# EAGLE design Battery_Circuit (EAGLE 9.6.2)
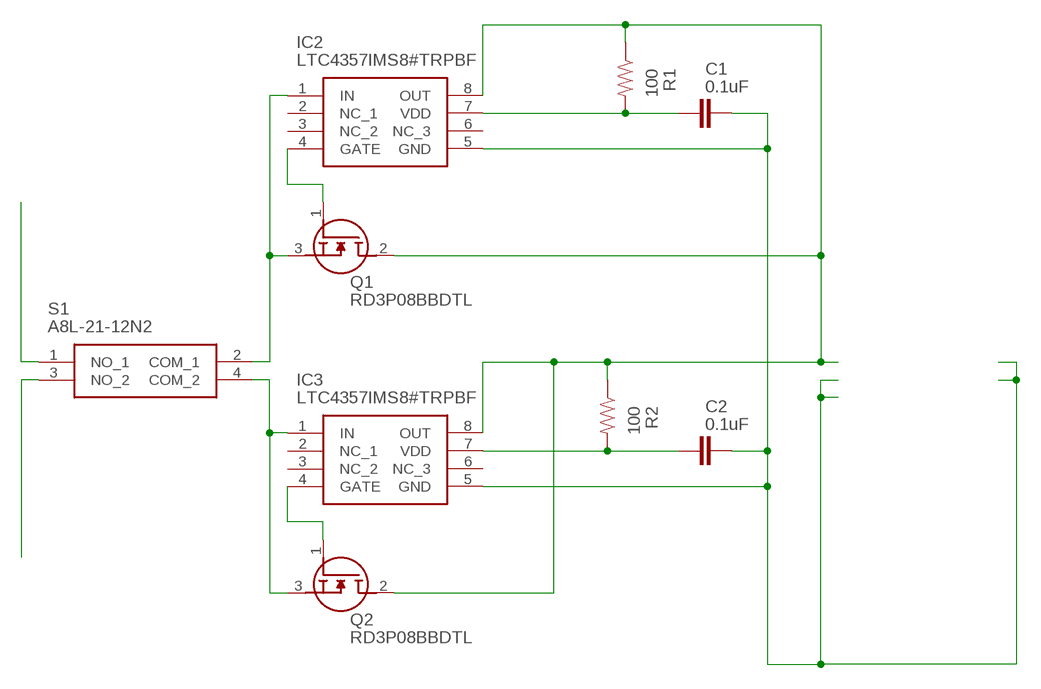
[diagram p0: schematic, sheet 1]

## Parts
C1  0.1uF  0.1UF-KIT-EZ-50V-20%  [CAP-PTH-SMALL-KIT]
C2  0.1uF  0.1UF-KIT-EZ-50V-20%  [CAP-PTH-SMALL-KIT]
IC2  LTC4357IMS8#TRPBF  [SOP65P490X110-8N]
IC3  LTC4357IMS8#TRPBF  [SOP65P490X110-8N]
Q1  RD3P08BBDTL  [RD3P175SNFRATL]
Q2  RD3P08BBDTL  [RD3P175SNFRATL]
R1  100  100OHM-HORIZ-1/4W-1%  [AXIAL-0.3]
R2  100  100OHM-HORIZ-1/4W-1%  [AXIAL-0.3]
S1  A8L-21-12N2  [A8L2112N2]

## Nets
N$1: IC2.1(IN) Q1.3(S) S1.2(COM_1)
N$2: IC2.4(GATE) Q1.1(G)
N$3: IC3.4(GATE) Q2.1(G)
N$4: S1.3(NO_2)
N$5: IC3.1(IN) Q2.3(S) S1.4(COM_2)
N$6: S1.1(NO_1)
N$7: C1.2 C2.2 IC2.5(GND) IC3.5(GND)
N$9: C1.1 IC2.7(VDD) R1.P$2
N$10: C2.1 IC3.7(VDD) R2.P$2
N$11: IC2.8(OUT) IC3.8(OUT) Q1.2(D) Q2.2(D) R1.P$1 R2.P$1
Unconnected: IC2.2(NC_1) IC2.3(NC_2) IC2.6(NC_3) IC3.2(NC_1) IC3.3(NC_2) IC3.6(NC_3)

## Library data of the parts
C1 C2 = SparkFun-Capacitors:0.1UF: 0.1µF ceramic capacitors; PROD_ID: CAP-08370
IC2 IC3 = SamacSys_Parts:LTC4357IMS8#TRPBF: Hot Swap Controller 1-CH 80V N-Channel Positive High Voltage Automotive 8-Pin MSOP T/R Source: Datasheet; ARROW_PART_NUMBER: LTC4357IMS8#TRPBF; ARROW_PRICE-STOCK: https://www.arrow.com/en/products/ltc4357ims8trpbf/analog-devices?region=nac; DESCRIPTION: Hot Swap Controller 1-CH 80V N-Channel Positive High Voltage Automotive 8-Pin MSOP T/R; HEIGHT: 1.1mm; MANUFACTURER_NAME: Analog Devices; MANUFACTURER_PART_NUMBER: LTC4357IMS8#TRPBF; MOUSER_PART_NUMBER: 584-LTC4357IMS8TRPBF; MOUSER_PRICE-STOCK: https://www.mouser.co.uk/ProductDetail/Analog-Devices/LTC4357IMS8TRPBF?qs=hVkxg5c3xu9xOCu4lpdF5Q%3D%3D
Q1 Q2 = SamacSys_Parts:RD3P08BBDTL: RD3P08BBDTL N-Channel MOSFET, 80 A, 100 V RD3P08BBD, 3-Pin DPAK ROHM Source: Datasheet; DESCRIPTION: RD3P08BBDTL N-Channel MOSFET, 80 A, 100 V RD3P08BBD, 3-Pin DPAK ROHM; HEIGHT: mm; MANUFACTURER_NAME: ROHM Semiconductor; MANUFACTURER_PART_NUMBER: RD3P08BBDTL; MOUSER_PART_NUMBER: 755-RD3P08BBDTL; MOUSER_PRICE-STOCK: https://www.mouser.co.uk/ProductDetail/ROHM-Semiconductor/RD3P08BBDTL?qs=qSfuJ%252Bfl%2Fd6NkJEicmek1A%3D%3D
R1 R2 = SparkFun-Resistors:100OHM: 100Ω resistor; PROD_ID: RES-12181
S1 = SamacSys_Parts:A8L-21-12N2: Rocker Switches ROCKER SWITCH Source: Datasheet; DESCRIPTION: Rocker Switches ROCKER SWITCH; HEIGHT: 22.1mm; MANUFACTURER_NAME: Omron Electronics; MANUFACTURER_PART_NUMBER: A8L-21-12N2; MOUSER_PART_NUMBER: 653-A8L-21-12N2; MOUSER_PRICE-STOCK: https://www.mouser.co.uk/ProductDetail/Omron-Electronics/A8L-21-12N2?qs=wE98CiVmOw76dmZWfHCJ3A%3D%3D

## Module DEWALT12V
Ports: 

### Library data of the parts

## Module 12V-5V_CONVERTER
Ports: IN-(in) IN+(in) OUT-(out) OUT+(out)

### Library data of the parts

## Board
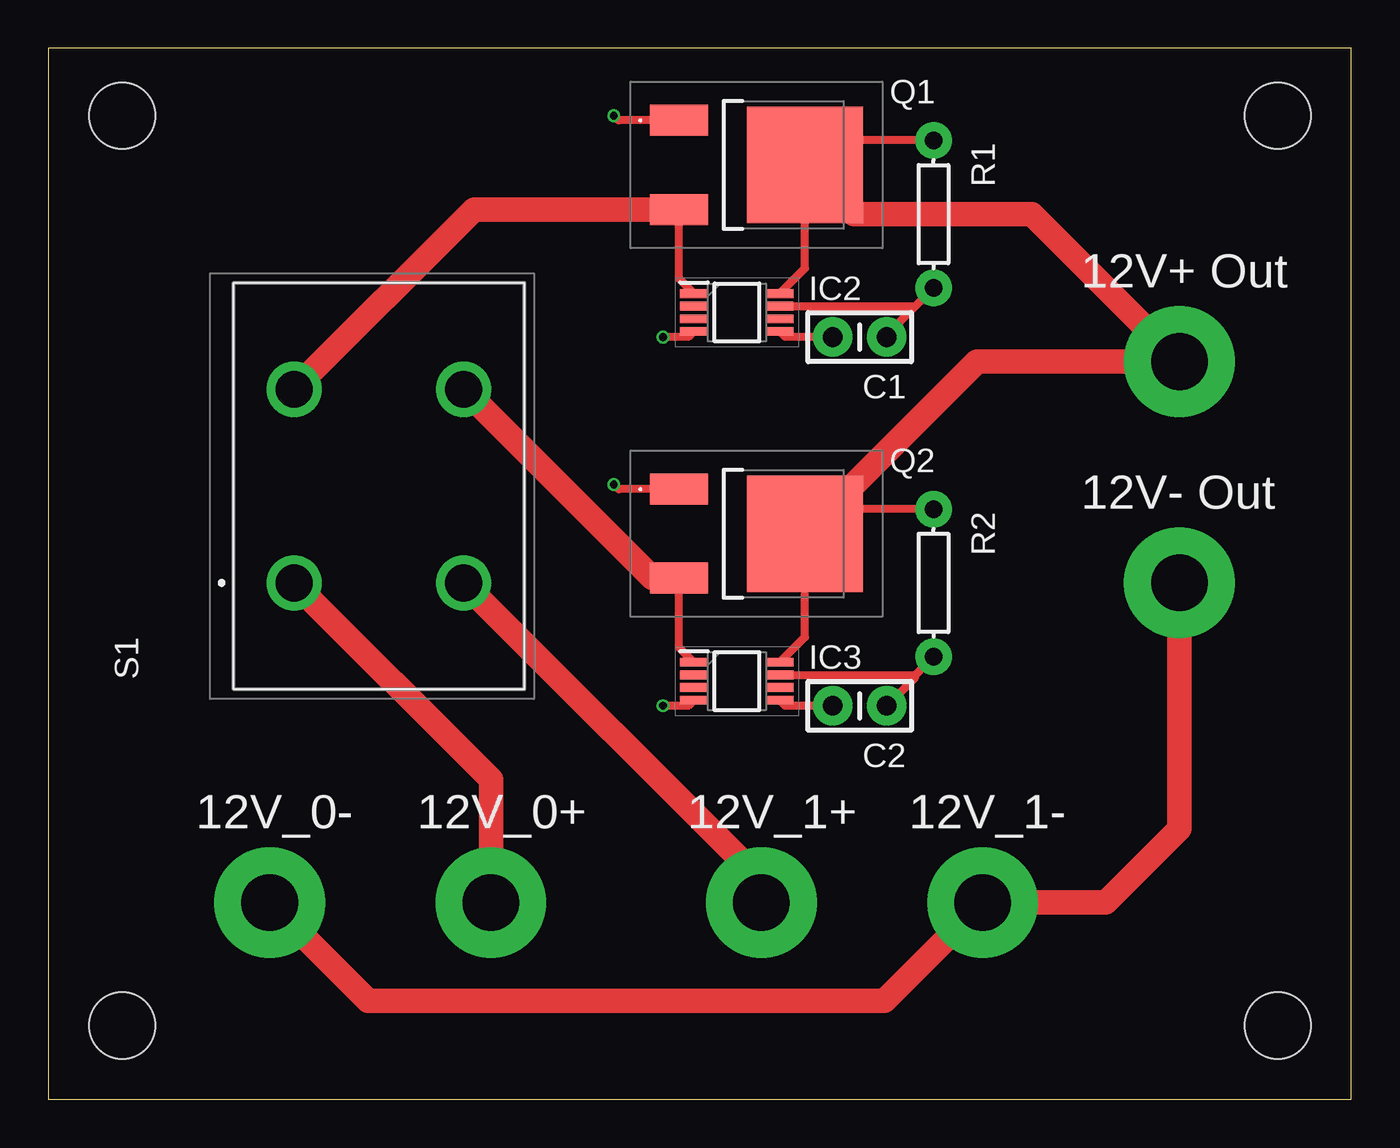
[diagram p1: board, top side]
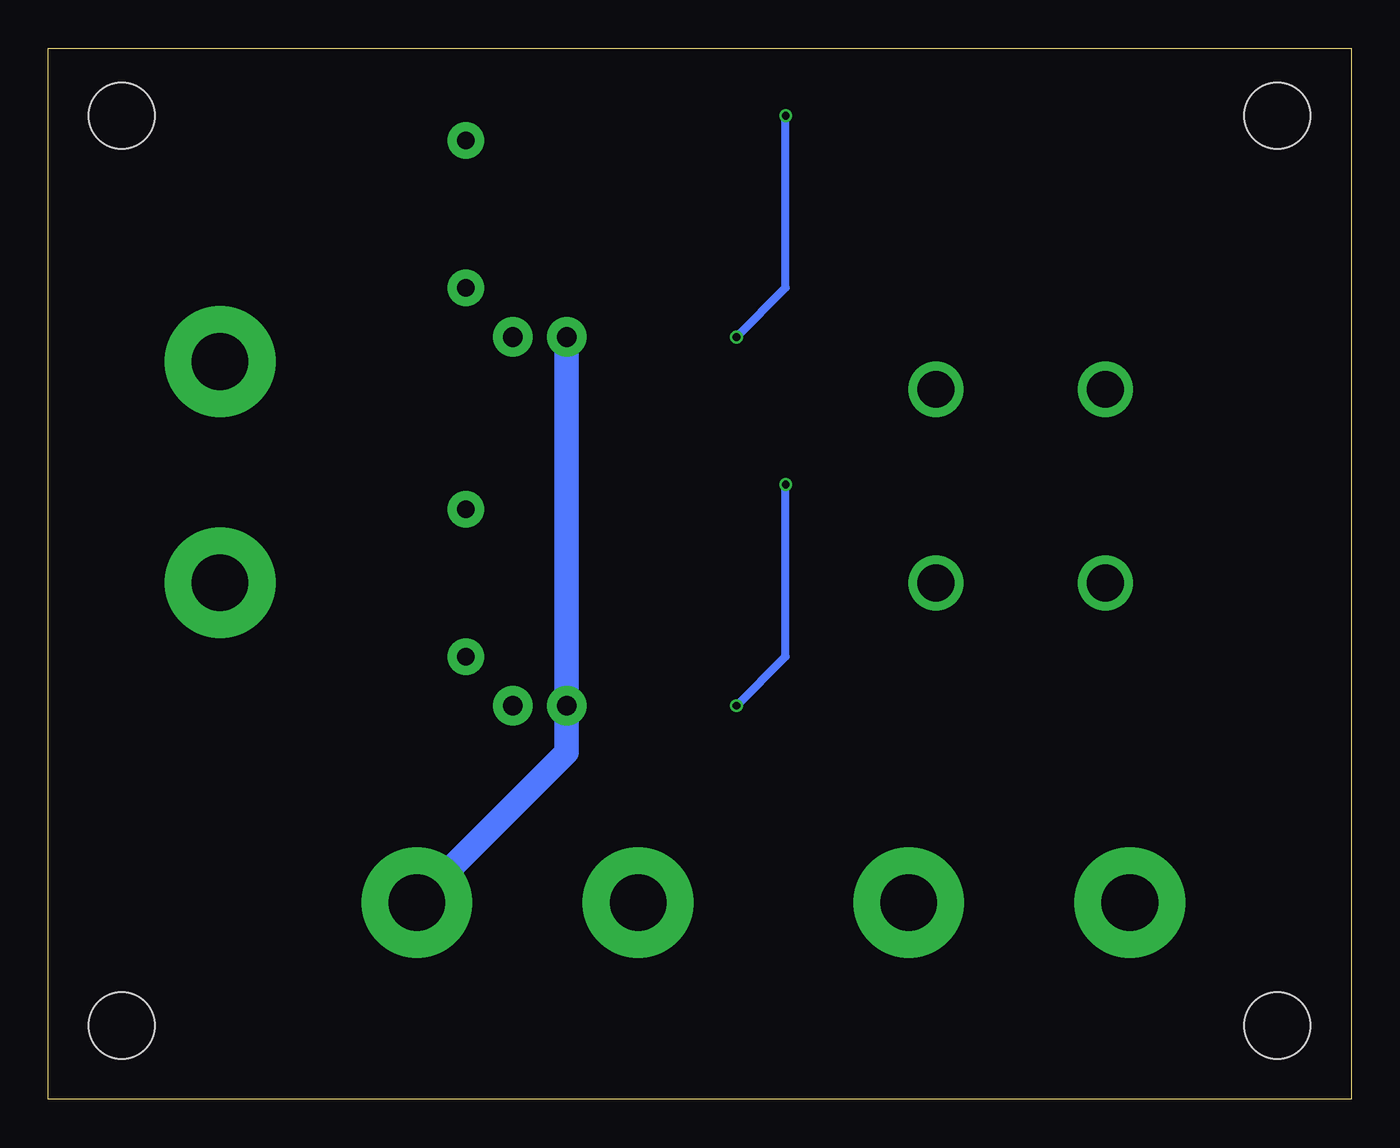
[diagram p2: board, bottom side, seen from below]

Size 67.29 x 54.28 mm. Coordinates in mm from the lower left corner, seen from the top.
Outline: 0,0 67.29,0 67.29,54.28 0,54.28 0,0
Copper layers (1*16): Top 0.035559375mm / dielectric 1.6mm / Bottom 0.035559375mm
Design rules "oshpark-2layer": minimum track width 6mil, minimum drill 10mil, track to track 6mil, track to pad 6mil, pad to pad 6mil, via to via 6mil, smd to smd 6mil, copper to edge 15mil, drill to drill 6mil, minimum pad ring 5mil, minimum via ring 5mil, stop-mask expansion 2.5mil, vias tented up to drill 0mil, thermal gap 10mil
Holes 3.43 mm at 3.81,3.81 3.81,50.8 63.5,50.8 63.5,3.81

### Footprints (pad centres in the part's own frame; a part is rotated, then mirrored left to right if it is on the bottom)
CAP-PTH-SMALL-KIT = drill 1.016 pad 2.032: 1 -1.397,0; 2 1.397,0
SOP65P490X110-8N = smd 1.425 x 0.45: 1 -2.212,0.975; 2 -2.212,0.325; 3 -2.212,-0.325; 4 -2.212,-0.975; 5 2.212,-0.975; 6 2.212,-0.325; 7 2.212,0.325; 8 2.212,0.975
RD3P175SNFRATL = smd 1.6 x 3: 1 -2.3,-4.25; 3 2.3,-4.25 | smd 6 x 6: 2 0,2.25
AXIAL-0.3 = drill 0.9 pad 1.88: P$1 -3.81,0; P$2 3.81,0
A8L2112N2 = drill 1.9 pad 2.85: 1 0,0; 2 10,0; 3 0,-8.75; 4 10,-8.75

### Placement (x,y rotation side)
C1  41.91,39.37 180 top
C2  41.91,20.32 180 top
IC2  35.56,40.64 0 top
IC3  35.56,21.59 0 top
Q1  36.83,48.26 270 top
Q2  36.83,29.21 270 top
R1  45.72,45.72 270 top
R2  45.72,26.67 270 top
S1  12.7,26.67 90 top

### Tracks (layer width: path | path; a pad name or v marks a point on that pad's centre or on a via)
N$1
  Top 0.406: IC2.1 32.58,42.38 Q1.3
  Top 1.27: S1.2 21.99,45.96 Q1.3
N$2  (via drill 0.4)
  Top 0.406: IC2.4 33.05,39.37 v31.75,39.37 | Q1.1 29.45,50.56 v29.21,50.8
  Bottom 0.406: v31.75,39.37 29.21,41.91 v29.21,50.8
N$3  (via drill 0.4)
  Top 0.406: IC3.4 33.05,20.32 v31.75,20.32 | Q2.1 29.45,31.51 v29.21,31.75
  Bottom 0.406: v31.75,20.32 29.21,22.86 v29.21,31.75
N$4  (via drill 2.92 pad 5.71)
  Top 1.27: v36.83,10.16 36.83,11.29 S1.3
N$5
  Top 0.406: IC3.1 32.58,23.33 Q2.3
  Top 1.27: S1.4 31.21,26.91 Q2.3
N$6  (via drill 2.92 pad 5.71)
  Top 1.27: S1.1 22.86,16.51 v22.86,10.16
N$7  (via drill 2.92 pad 5.71)
  Top 0.406: C2.2 38.07,20.32 IC3.5 | C1.2 38.07,39.37 IC2.5
  Top 1.27: v58.42,26.67 58.42,13.97 54.61,10.16 v48.26,10.16 43.18,5.08 16.51,5.08 v11.43,10.16
  Bottom 1.27: C1.2 C2.2 40.51,17.91 v48.26,10.16
N$9
  Top 0.406: IC2.7 44.77,40.97 | 44.77,40.97 R1.P$2 | C1.1 43.31,39.5 44.77,40.97
N$10
  Top 0.406: IC3.7 44.77,21.91 | 44.77,21.91 R2.P$2 | C2.1 44.77,21.79 44.77,21.91
N$11  (via drill 2.92 pad 5.71)
  Top 0.406: IC3.8 39.08,23.87 Q2.2 40.35,30.48 R2.P$1 | IC2.8 39.08,42.92 Q1.2 40.35,49.53 R1.P$1
  Top 1.27: Q1.2 41.62,45.72 50.8,45.72 v58.42,38.1 47.97,38.1 Q2.2

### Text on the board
tNames: 12V+ Out | 12V- Out | 12V_0- | 12V_0+ | 12V_1+ | 12V_1-

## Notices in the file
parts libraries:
SparkFun-Resistors: Licensing: Creative Commons ShareAlike 4.0 International - https://creativecommons.org/licenses/by-sa/4.0
